| IBIS file stm32u535_545_ufbga100.ibs
[IBIS ver] 4.2
[File name] stm32u535_545_ufbga100.ibs
[File Rev] rev1.0
[Date]  11-09-2023
[Source] Data Created at STMicroelectronics
[Notes]  File originated from ELDO simulations.
[Disclaimer]  This information is for modeling purpose only and is
   not guaranteed. The information is subject to change without
   notice.
[Copyright] Copyright 2023 STMicroelectronics Inc.
|   Component stm32u535_545_ufbga100
[Component] stm32u535_545_ufbga100
[Manufacturer] STMicroelectronics
[Package]
| variable   typ   min   max
R_pkg  0  NA  NA
L_pkg  0  NA  NA
C_pkg  0  NA  NA
[Pin]   signal_name   model_name
A1  PE3  io8_100m_hslv_tamp_ft
A2  PE1  io8_100m_hslv_ft
A3  PB8  io8_100m_hslv_i2c_ft
A4  PH3-BOOT0  io8_100m_ft
A5  PD7  io8_100m_hslv_ft
A6  PD5  io8_100m_hslv_ft
A7  PB4  io8_100m_i2c_ft
A8  PB3  io8_100m_i2c_ft
A9  PA15  io8_100m_ft
A10  PA14  io8_100m_ft
A11  PA13  io8_100m_ft
A12  PA12  io8_usb_ft
B1  PE4  io8_100m_hslv_tamp_ft
B2  PE2  io8_100m_hslv_ft
B3  PB9  io8_100m_hslv_i2c_ft
B4  PB7  io8_166m_hslv_i2c_ft
B5  PB6  io8_100m_i2c_ft
B6  PD6  io8_166m_hslv_ft
B7  PD4  io8_100m_hslv_ft
B8  PD3  io8_166m_hslv_ft
B9  PD1  io8_100m_hslv_ft
B10  PC12  io8_166m_hslv_ft
B11  PC10  io8_100m_hslv_ft
B12  PA11  io8_usb_ft
C1  PC13  io8_100m_ft_v33
C2  PE5  io8_100m_hslv_tamp_ft
C3  PE0  io8_100m_hslv_ft
C4  VDD  power
C5  PB5  io8_166m_hslv_ft
C8  PD2  io8_100m_hslv_ft
C9  PD0  io8_100m_hslv_ft
C10  PC11  io8_100m_hslv_ft
C11  VDDUSB  power
C12  PA10  io8_100m_ft
D1  PC14-OSC32_IN  io8_100m_tamp_ft
D2  PE6  io8_100m_hslv_tamp_ft
D3  VSS  gnd
D10  PA9  io8_100m_ft
D11  PA8  io8_166m_hslv_ft
D12  PC9  io8_100m_hslv_ft
E1  PC15-OSC32_OUT  io8_100m_tamp_ft
E2  VBAT  power
E3  VSS  gnd
E10  PC8  io8_100m_hslv_ft
E11  PC7  io8_100m_hslv_ft
E12  PC6  io8_100m_hslv_ft
F1  PH0-OSC_IN   io8_100m_ft
F2  VSS  gnd
F11  VSS  gnd
F12  VSS  gnd
G1  PH1-OSC_OUT   io8_100m_ft
G2  VDD  power
G11  VDD  power
G12  VDD  power
H1  PC0  io8_100m_hslv_i2c_ft
H2  NRST  nc
H3  VDD  power
H10  PD15  io8_100m_hslv_ft
H11  PD14  io8_100m_hslv_ft
H12  PD13  io8_100m_hslv_i2c_ft
J1  VSSA  nc
J2  PC1  io8_166m_hslv_i2c_ft
J3  PC2  io8_100m_hslv_ft
J10  PD12  io8_100m_hslv_i2c_ft
J11  PD11  io8_100m_hslv_ft
J12  PD10  io8_100m_hslv_ft
K1  VREFM  nc
K2  PC3  io8_100m_hslv_ft
K3  PA2  io8_100m_hslv_ft
K4  PA5  io8_100m_ft
K5  PC4  io8_100m_hslv_ft
K8  PD9  io8_100m_hslv_ft
K9  PD8  io8_100m_hslv_ft
K10  PB15  io8_100m_ft
K11  PB14  io8_100m_i2c_ft
K12  PB13  io8_100m_i2c_ft
L1  VREFP  nc
L2  PA0  io8_100m_hslv_tamp_ft
L3  PA3  io8_166m_hslv_ft
L4  PA6  io8_100m_hslv_ft
L5  PC5  io8_100m_tamp_ft
L6  PB2  io8_100m_hslv_tamp_ft
L7  PE8  io8_100m_hslv_ft
L8  PE10  io8_166m_hslv_ft
L9  PE12  io8_100m_hslv_ft
L10  PB10  io8_166m_hslv_i2c_ft
L11  VCAP  nc
L12  PB12  io8_166m_hslv_ft
M1  VDDA  power
M2  PA1  io8_100m_hslv_tamp_ft
M3  PA4  io8_100m_hslv_ft
M4  PA7  io8_100m_hslv_i2c_ft
M5  PB0  io8_100m_hslv_ft
M6  PB1  io8_100m_hslv_ft
M7  PE7  io8_100m_hslv_ft
M8  PE9  io8_166m_hslv_ft
M9  PE11  io8_100m_hslv_ft
M10  PE13  io8_100m_hslv_ft
M11  PE14  io8_100m_hslv_ft
M12  PE15  io8_100m_hslv_ft
[Package Model]   455-ufbga-7x7-100-ldo-100mhz-230421
[Pin Mapping]   pulldown_ref   pullup_ref   | Comment
A1  gndio  vddiom
A2  gndio  vddiom
A3  gndio  vddiom
A4  gndio  vddiom
A5  gndio  vddiom
A6  gndio  vddiom
A7  gndio  vddiom
A8  gndio  vddiom
A9  gndio  vddiom
A10  gndio  vddiom
A11  gndio  vddiom  | Depending on IO usage
| A11  gndio  vddusb  | Depending on IO usage
A12  gndio  vddiom  | Depending on IO usage
| A12  gndio  vddusb  | Depending on IO usage
B1  gndio  vddiom
B2  gndio  vddiom
B3  gndio  vddiom
B4  gndio  vddiom
B5  gndio  vddiom
B6  gndio  vddiom
B7  gndio  vddiom
B8  gndio  vddiom
B9  gndio  vddiom
B10  gndio  vddiom
B11  gndio  vddiom
B12  gndio  vddiom  | Depending on IO usage
| B12  gndio  vddusb  | Depending on IO usage
C1  gndio  vddiom  | Depending on IO usage
| C1  gndio  vsw  | Depending on IO usage
C2  gndio  vddiom
C3  gndio  vddiom
C4  nc  vddiom
C5  gndio  vddiom
C8  gndio  vddiom
C9  gndio  vddiom
C10  gndio  vddiom
C11  nc  vddusb
C12  gndio  vddiom  | Depending on IO usage
| C12  gndio  vddusb  | Depending on IO usage
D1  gndio  vddiom  | Depending on IO usage
| D1  gndio  vsw  | Depending on IO usage
D2  gndio  vddiom
D3  gndio  nc
D10  gndio  vddiom  | Depending on IO usage
| D10  gndio  vddusb  | Depending on IO usage
D11  gndio  vddiom
D12  gndio  vddiom
E1  gndio  vddiom  | Depending on IO usage
| E1  gndio  vsw  | Depending on IO usage
E2  nc  vsw
E3  gndio  nc
E10  gndio  vddiom
E11  gndio  vddiom
E12  gndio  vddiom
F1  gndio  vddiom
F2  gndio  nc
F11  gndio  nc
F12  gndio  nc
G1  gndio  vddiom
G2  nc  vddiom
G11  nc  vddiom
G12  nc  vddiom
H1  gndio  vddiom
H2  nc   nc
H3  nc  vddiom
H10  gndio  vddiom
H11  gndio  vddiom
H12  gndio  vddiom
J1  nc  nc
J2  gndio  vddiom
J3  gndio  vddiom
J10  gndio  vddiom
J11  gndio  vddiom
J12  gndio  vddiom
K1  nc  nc
K2  gndio  vddiom
K3  gndio  vddiom
K4  gndio  vddiom
K5  gndio  vddiom
K8  gndio  vddiom
K9  gndio  vddiom
K10  gndio  vddiom
K11  gndio  vddiom
K12  gndio  vddiom
L1  nc  nc
L2  gndio  vddiom
L3  gndio  vddiom
L4  gndio  vddiom
L5  gndio  vddiom
L6  gndio  vddiom
L7  gndio  vddiom
L8  gndio  vddiom
L9  gndio  vddiom
L10  gndio  vddiom
L11  nc  nc
L12  gndio  vddiom
M1  nc  vddiom
M2  gndio  vddiom
M3  gndio  vddiom
M4  gndio  vddiom
M5  gndio  vddiom
M6  gndio  vddiom
M7  gndio  vddiom
M8  gndio  vddiom
M9  gndio  vddiom
M10  gndio  vddiom
M11  gndio  vddiom
M12  gndio  vddiom
[Model Selector] io8_100m_ft
io8_100m_ft_hs_1v2  "IO8_FT 100MHz high speed @ 1.2V"
io8_100m_ft_fs_1v2  "IO8_FT 100MHz fast speed @ 1.2V"
io8_100m_ft_fs_pd_1v2  "IO8_FT 100MHz fast speed @ 1.2V pulldown"
io8_100m_ft_ms_1v2  "IO8_FT 100MHz med speed @ 1.2V"
io8_100m_ft_ms_pd_1v2  "IO8_FT 100MHz med speed @ 1.2V pulldown"
io8_100m_ft_ls_1v2  "IO8_FT 100MHz low speed @ 1.2V"
io8_100m_ft_ls_pd_1v2  "IO8_FT 100MHz low speed @ 1.2V pulldown"
io8_100m_ft_hs_1v8  "IO8_FT 100MHz high speed @ 1.8V"
io8_100m_ft_hs_pd_1v8  "IO8_FT 100MHz high speed @ 1.8V pulldown"
io8_100m_ft_fs_1v8  "IO8_FT 100MHz fast speed @ 1.8V"
io8_100m_ft_fs_pd_1v8  "IO8_FT 100MHz fast speed @ 1.8V pulldown"
io8_100m_ft_ms_1v8  "IO8_FT 100MHz med speed @ 1.8V"
io8_100m_ft_ms_pd_1v8  "IO8_FT 100MHz med speed @ 1.8V pulldown"
io8_100m_ft_ls_1v8  "IO8_FT 100MHz low speed @ 1.8V"
io8_100m_ft_ls_pd_1v8  "IO8_FT 100MHz low speed @ 1.8V pulldown"
io8_100m_ft_hs_3v3  "IO8_FT 100MHz high speed @ 3.3V"
io8_100m_ft_hs_pd_3v3  "IO8_FT 100MHz high speed @ 3.3V pulldown"
io8_100m_ft_fs_3v3  "IO8_FT 100MHz fast speed @ 3.3V"
io8_100m_ft_fs_pd_3v3  "IO8_FT 100MHz fast speed @ 3.3V pulldown"
io8_100m_ft_ms_3v3  "IO8_FT 100MHz med speed @ 3.3V"
io8_100m_ft_ms_pd_3v3  "IO8_FT 100MHz med speed @ 3.3V pulldown"
io8_100m_ft_ls_3v3  "IO8_FT 100MHz low speed @ 3.3V"
io8_100m_ft_ls_pd_3v3  "IO8_FT 100MHz low speed @ 3.3V pulldown"
[Model Selector] io8_100m_hslv_ft
io8_100m_ft_hs_1v2  "IO8_FT 100MHz high speed @ 1.2V"
io8_100m_ft_hs_pu_1v2  "IO8_FT 100MHz high speed @ 1.2V pullup"
io8_100m_ft_hs_pd_1v2  "IO8_FT 100MHz high speed @ 1.2V pulldown"
io8_100m_ft_fs_1v2  "IO8_FT 100MHz fast speed @ 1.2V"
io8_100m_ft_fs_pu_1v2  "IO8_FT 100MHz fast speed @ 1.2V pullup"
io8_100m_ft_fs_pd_1v2  "IO8_FT 100MHz fast speed @ 1.2V pulldown"
io8_100m_ft_ms_1v2  "IO8_FT 100MHz med speed @ 1.2V"
io8_100m_ft_ms_pu_1v2  "IO8_FT 100MHz med speed @ 1.2V pullup"
io8_100m_ft_ms_pd_1v2  "IO8_FT 100MHz med speed @ 1.2V pulldown"
io8_100m_ft_ls_1v2  "IO8_FT 100MHz low speed @ 1.2V"
io8_100m_ft_ls_pu_1v2  "IO8_FT 100MHz low speed @ 1.2V pullup"
io8_100m_ft_ls_pd_1v2  "IO8_FT 100MHz low speed @ 1.2V pulldown"
io8_100m_ft_hs_1v8  "IO8_FT 100MHz high speed @ 1.8V"
io8_100m_ft_hs_pu_1v8  "IO8_FT 100MHz high speed @ 1.8V pullup"
io8_100m_ft_hs_pd_1v8  "IO8_FT 100MHz high speed @ 1.8V pulldown"
io8_100m_ft_fs_1v8  "IO8_FT 100MHz fast speed @ 1.8V"
io8_100m_ft_fs_pu_1v8  "IO8_FT 100MHz fast speed @ 1.8V pullup"
io8_100m_ft_fs_pd_1v8  "IO8_FT 100MHz fast speed @ 1.8V pulldown"
io8_100m_ft_ms_1v8  "IO8_FT 100MHz med speed @ 1.8V"
io8_100m_ft_ms_pu_1v8  "IO8_FT 100MHz med speed @ 1.8V pullup"
io8_100m_ft_ms_pd_1v8  "IO8_FT 100MHz med speed @ 1.8V pulldown"
io8_100m_ft_ls_1v8  "IO8_FT 100MHz low speed @ 1.8V"
io8_100m_ft_ls_pu_1v8  "IO8_FT 100MHz low speed @ 1.8V pullup"
io8_100m_ft_ls_pd_1v8  "IO8_FT 100MHz low speed @ 1.8V pulldown"
io8_100m_ft_hs_3v3  "IO8_FT 100MHz high speed @ 3.3V"
io8_100m_ft_hs_pu_3v3  "IO8_FT 100MHz high speed @ 3.3V pullup"
io8_100m_ft_hs_pd_3v3  "IO8_FT 100MHz high speed @ 3.3V pulldown"
io8_100m_ft_fs_3v3  "IO8_FT 100MHz fast speed @ 3.3V"
io8_100m_ft_fs_pu_3v3  "IO8_FT 100MHz fast speed @ 3.3V pullup"
io8_100m_ft_fs_pd_3v3  "IO8_FT 100MHz fast speed @ 3.3V pulldown"
io8_100m_ft_ms_3v3  "IO8_FT 100MHz med speed @ 3.3V"
io8_100m_ft_ms_pu_3v3  "IO8_FT 100MHz med speed @ 3.3V pullup"
io8_100m_ft_ms_pd_3v3  "IO8_FT 100MHz med speed @ 3.3V pulldown"
io8_100m_ft_ls_3v3  "IO8_FT 100MHz low speed @ 3.3V"
io8_100m_ft_ls_pu_3v3  "IO8_FT 100MHz low speed @ 3.3V pullup"
io8_100m_ft_ls_pd_3v3  "IO8_FT 100MHz low speed @ 3.3V pulldown"
io8_100m_hslv_ft_hs_1v2  "IO8_FT 100MHz HSLV high speed @ 1.2V"
io8_100m_hslv_ft_hs_pu_1v2  "IO8_FT 100MHz HSLV high speed @ 1.2V pullup"
io8_100m_hslv_ft_hs_pd_1v2  "IO8_FT 100MHz HSLV high speed @ 1.2V pulldown"
io8_100m_hslv_ft_fs_1v2  "IO8_FT 100MHz HSLV fast speed @ 1.2V"
io8_100m_hslv_ft_fs_pu_1v2  "IO8_FT 100MHz HSLV fast speed @ 1.2V pullup"
io8_100m_hslv_ft_fs_pd_1v2  "IO8_FT 100MHz HSLV fast speed @ 1.2V pulldown"
io8_100m_hslv_ft_ms_1v2  "IO8_FT 100MHz HSLV med speed @ 1.2V"
io8_100m_hslv_ft_ms_pu_1v2  "IO8_FT 100MHz HSLV med speed @ 1.2V pullup"
io8_100m_hslv_ft_ms_pd_1v2  "IO8_FT 100MHz HSLV med speed @ 1.2V pulldown"
io8_100m_hslv_ft_ls_1v2  "IO8_FT 100MHz HSLV low speed @ 1.2V"
io8_100m_hslv_ft_ls_pu_1v2  "IO8_FT 100MHz HSLV low speed @ 1.2V pullup"
io8_100m_hslv_ft_ls_pd_1v2  "IO8_FT 100MHz HSLV low speed @ 1.2V pulldown"
io8_100m_hslv_ft_hs_1v8  "IO8_FT 100MHz HSLV high speed @ 1.8V"
io8_100m_hslv_ft_hs_pu_1v8  "IO8_FT 100MHz HSLV high speed @ 1.8V pullup"
io8_100m_hslv_ft_hs_pd_1v8  "IO8_FT 100MHz HSLV high speed @ 1.8V pulldown"
io8_100m_hslv_ft_fs_1v8  "IO8_FT 100MHz HSLV fast speed @ 1.8V"
io8_100m_hslv_ft_fs_pu_1v8  "IO8_FT 100MHz HSLV fast speed @ 1.8V pullup"
io8_100m_hslv_ft_fs_pd_1v8  "IO8_FT 100MHz HSLV fast speed @ 1.8V pulldown"
io8_100m_hslv_ft_ms_1v8  "IO8_FT 100MHz HSLV med speed @ 1.8V"
io8_100m_hslv_ft_ms_pu_1v8  "IO8_FT 100MHz HSLV med speed @ 1.8V pullup"
io8_100m_hslv_ft_ms_pd_1v8  "IO8_FT 100MHz HSLV med speed @ 1.8V pulldown"
io8_100m_hslv_ft_ls_1v8  "IO8_FT 100MHz HSLV low speed @ 1.8V"
io8_100m_hslv_ft_ls_pu_1v8  "IO8_FT 100MHz HSLV low speed @ 1.8V pullup"
io8_100m_hslv_ft_ls_pd_1v8  "IO8_FT 100MHz HSLV low speed @ 1.8V pulldown"
io8_100m_hslv_ft_hs_2v5  "IO8_FT 100MHz HSLV high speed @ 2.5V"
io8_100m_hslv_ft_hs_pu_2v5  "IO8_FT 100MHz HSLV high speed @ 2.5V pullup"
io8_100m_hslv_ft_hs_pd_2v5  "IO8_FT 100MHz HSLV high speed @ 2.5V pulldown"
io8_100m_hslv_ft_fs_2v5  "IO8_FT 100MHz HSLV fast speed @ 2.5V"
io8_100m_hslv_ft_fs_pu_2v5  "IO8_FT 100MHz HSLV fast speed @ 2.5V pullup"
io8_100m_hslv_ft_fs_pd_2v5  "IO8_FT 100MHz HSLV fast speed @ 2.5V pulldown"
io8_100m_hslv_ft_ms_2v5  "IO8_FT 100MHz HSLV med speed @ 2.5V"
io8_100m_hslv_ft_ms_pu_2v5  "IO8_FT 100MHz HSLV med speed @ 2.5V pullup"
io8_100m_hslv_ft_ms_pd_2v5  "IO8_FT 100MHz HSLV med speed @ 2.5V pulldown"
io8_100m_hslv_ft_ls_2v5  "IO8_FT 100MHz HSLV low speed @ 2.5V"
io8_100m_hslv_ft_ls_pu_2v5  "IO8_FT 100MHz HSLV low speed @ 2.5V pullup"
io8_100m_hslv_ft_ls_pd_2v5  "IO8_FT 100MHz HSLV low speed @ 2.5V pulldown"
[Model Selector] io8_100m_hslv_i2c_ft
io8_100m_ft_hs_1v2  "IO8_FT 100MHz high speed @ 1.2V"
io8_100m_ft_hs_pu_1v2  "IO8_FT 100MHz high speed @ 1.2V pullup"
io8_100m_ft_hs_pd_1v2  "IO8_FT 100MHz high speed @ 1.2V pulldown"
io8_100m_ft_fs_1v2  "IO8_FT 100MHz fast speed @ 1.2V"
io8_100m_ft_fs_pu_1v2  "IO8_FT 100MHz fast speed @ 1.2V pullup"
io8_100m_ft_fs_pd_1v2  "IO8_FT 100MHz fast speed @ 1.2V pulldown"
io8_100m_ft_ms_1v2  "IO8_FT 100MHz med speed @ 1.2V"
io8_100m_ft_ms_pu_1v2  "IO8_FT 100MHz med speed @ 1.2V pullup"
io8_100m_ft_ms_pd_1v2  "IO8_FT 100MHz med speed @ 1.2V pulldown"
io8_100m_ft_ls_1v2  "IO8_FT 100MHz low speed @ 1.2V"
io8_100m_ft_ls_pu_1v2  "IO8_FT 100MHz low speed @ 1.2V pullup"
io8_100m_ft_ls_pd_1v2  "IO8_FT 100MHz low speed @ 1.2V pulldown"
io8_100m_ft_hs_1v8  "IO8_FT 100MHz high speed @ 1.8V"
io8_100m_ft_hs_pu_1v8  "IO8_FT 100MHz high speed @ 1.8V pullup"
io8_100m_ft_hs_pd_1v8  "IO8_FT 100MHz high speed @ 1.8V pulldown"
io8_100m_ft_fs_1v8  "IO8_FT 100MHz fast speed @ 1.8V"
io8_100m_ft_fs_pu_1v8  "IO8_FT 100MHz fast speed @ 1.8V pullup"
io8_100m_ft_fs_pd_1v8  "IO8_FT 100MHz fast speed @ 1.8V pulldown"
io8_100m_ft_ms_1v8  "IO8_FT 100MHz med speed @ 1.8V"
io8_100m_ft_ms_pu_1v8  "IO8_FT 100MHz med speed @ 1.8V pullup"
io8_100m_ft_ms_pd_1v8  "IO8_FT 100MHz med speed @ 1.8V pulldown"
io8_100m_ft_ls_1v8  "IO8_FT 100MHz low speed @ 1.8V"
io8_100m_ft_ls_pu_1v8  "IO8_FT 100MHz low speed @ 1.8V pullup"
io8_100m_ft_ls_pd_1v8  "IO8_FT 100MHz low speed @ 1.8V pulldown"
io8_100m_ft_hs_3v3  "IO8_FT 100MHz high speed @ 3.3V"
io8_100m_ft_hs_pu_3v3  "IO8_FT 100MHz high speed @ 3.3V pullup"
io8_100m_ft_hs_pd_3v3  "IO8_FT 100MHz high speed @ 3.3V pulldown"
io8_100m_ft_fs_3v3  "IO8_FT 100MHz fast speed @ 3.3V"
io8_100m_ft_fs_pu_3v3  "IO8_FT 100MHz fast speed @ 3.3V pullup"
io8_100m_ft_fs_pd_3v3  "IO8_FT 100MHz fast speed @ 3.3V pulldown"
io8_100m_ft_ms_3v3  "IO8_FT 100MHz med speed @ 3.3V"
io8_100m_ft_ms_pu_3v3  "IO8_FT 100MHz med speed @ 3.3V pullup"
io8_100m_ft_ms_pd_3v3  "IO8_FT 100MHz med speed @ 3.3V pulldown"
io8_100m_ft_ls_3v3  "IO8_FT 100MHz low speed @ 3.3V"
io8_100m_ft_ls_pu_3v3  "IO8_FT 100MHz low speed @ 3.3V pullup"
io8_100m_ft_ls_pd_3v3  "IO8_FT 100MHz low speed @ 3.3V pulldown"
io8_100m_hslv_ft_hs_1v2  "IO8_FT 100MHz HSLV high speed @ 1.2V"
io8_100m_hslv_ft_hs_pu_1v2  "IO8_FT 100MHz HSLV high speed @ 1.2V pullup"
io8_100m_hslv_ft_hs_pd_1v2  "IO8_FT 100MHz HSLV high speed @ 1.2V pulldown"
io8_100m_hslv_ft_fs_1v2  "IO8_FT 100MHz HSLV fast speed @ 1.2V"
io8_100m_hslv_ft_fs_pu_1v2  "IO8_FT 100MHz HSLV fast speed @ 1.2V pullup"
io8_100m_hslv_ft_fs_pd_1v2  "IO8_FT 100MHz HSLV fast speed @ 1.2V pulldown"
io8_100m_hslv_ft_ms_1v2  "IO8_FT 100MHz HSLV med speed @ 1.2V"
io8_100m_hslv_ft_ms_pu_1v2  "IO8_FT 100MHz HSLV med speed @ 1.2V pullup"
io8_100m_hslv_ft_ms_pd_1v2  "IO8_FT 100MHz HSLV med speed @ 1.2V pulldown"
io8_100m_hslv_ft_ls_1v2  "IO8_FT 100MHz HSLV low speed @ 1.2V"
io8_100m_hslv_ft_ls_pu_1v2  "IO8_FT 100MHz HSLV low speed @ 1.2V pullup"
io8_100m_hslv_ft_ls_pd_1v2  "IO8_FT 100MHz HSLV low speed @ 1.2V pulldown"
io8_100m_hslv_ft_hs_1v8  "IO8_FT 100MHz HSLV high speed @ 1.8V"
io8_100m_hslv_ft_hs_pu_1v8  "IO8_FT 100MHz HSLV high speed @ 1.8V pullup"
io8_100m_hslv_ft_hs_pd_1v8  "IO8_FT 100MHz HSLV high speed @ 1.8V pulldown"
io8_100m_hslv_ft_fs_1v8  "IO8_FT 100MHz HSLV fast speed @ 1.8V"
io8_100m_hslv_ft_fs_pu_1v8  "IO8_FT 100MHz HSLV fast speed @ 1.8V pullup"
io8_100m_hslv_ft_fs_pd_1v8  "IO8_FT 100MHz HSLV fast speed @ 1.8V pulldown"
io8_100m_hslv_ft_ms_1v8  "IO8_FT 100MHz HSLV med speed @ 1.8V"
io8_100m_hslv_ft_ms_pu_1v8  "IO8_FT 100MHz HSLV med speed @ 1.8V pullup"
io8_100m_hslv_ft_ms_pd_1v8  "IO8_FT 100MHz HSLV med speed @ 1.8V pulldown"
io8_100m_hslv_ft_ls_1v8  "IO8_FT 100MHz HSLV low speed @ 1.8V"
io8_100m_hslv_ft_ls_pu_1v8  "IO8_FT 100MHz HSLV low speed @ 1.8V pullup"
io8_100m_hslv_ft_ls_pd_1v8  "IO8_FT 100MHz HSLV low speed @ 1.8V pulldown"
io8_100m_hslv_ft_hs_2v5  "IO8_FT 100MHz HSLV high speed @ 2.5V"
io8_100m_hslv_ft_hs_pu_2v5  "IO8_FT 100MHz HSLV high speed @ 2.5V pullup"
io8_100m_hslv_ft_hs_pd_2v5  "IO8_FT 100MHz HSLV high speed @ 2.5V pulldown"
io8_100m_hslv_ft_fs_2v5  "IO8_FT 100MHz HSLV fast speed @ 2.5V"
io8_100m_hslv_ft_fs_pu_2v5  "IO8_FT 100MHz HSLV fast speed @ 2.5V pullup"
io8_100m_hslv_ft_fs_pd_2v5  "IO8_FT 100MHz HSLV fast speed @ 2.5V pulldown"
io8_100m_hslv_ft_ms_2v5  "IO8_FT 100MHz HSLV med speed @ 2.5V"
io8_100m_hslv_ft_ms_pu_2v5  "IO8_FT 100MHz HSLV med speed @ 2.5V pullup"
io8_100m_hslv_ft_ms_pd_2v5  "IO8_FT 100MHz HSLV med speed @ 2.5V pulldown"
io8_100m_hslv_ft_ls_2v5  "IO8_FT 100MHz HSLV low speed @ 2.5V"
io8_100m_hslv_ft_ls_pu_2v5  "IO8_FT 100MHz HSLV low speed @ 2.5V pullup"
io8_100m_hslv_ft_ls_pd_2v5  "IO8_FT 100MHz HSLV low speed @ 2.5V pulldown"
[Model Selector] io8_100m_hslv_tamp_ft
io8_100m_ft_hs_1v2  "IO8_FT 100MHz high speed @ 1.2V"
io8_100m_ft_hs_pu_1v2  "IO8_FT 100MHz high speed @ 1.2V pullup"
io8_100m_ft_hs_pd_1v2  "IO8_FT 100MHz high speed @ 1.2V pulldown"
io8_100m_ft_fs_1v2  "IO8_FT 100MHz fast speed @ 1.2V"
io8_100m_ft_fs_pu_1v2  "IO8_FT 100MHz fast speed @ 1.2V pullup"
io8_100m_ft_fs_pd_1v2  "IO8_FT 100MHz fast speed @ 1.2V pulldown"
io8_100m_ft_ms_1v2  "IO8_FT 100MHz med speed @ 1.2V"
io8_100m_ft_ms_pu_1v2  "IO8_FT 100MHz med speed @ 1.2V pullup"
io8_100m_ft_ms_pd_1v2  "IO8_FT 100MHz med speed @ 1.2V pulldown"
io8_100m_ft_ls_1v2  "IO8_FT 100MHz low speed @ 1.2V"
io8_100m_ft_ls_pu_1v2  "IO8_FT 100MHz low speed @ 1.2V pullup"
io8_100m_ft_ls_pd_1v2  "IO8_FT 100MHz low speed @ 1.2V pulldown"
io8_100m_ft_hs_1v8  "IO8_FT 100MHz high speed @ 1.8V"
io8_100m_ft_hs_pu_1v8  "IO8_FT 100MHz high speed @ 1.8V pullup"
io8_100m_ft_hs_pd_1v8  "IO8_FT 100MHz high speed @ 1.8V pulldown"
io8_100m_ft_fs_1v8  "IO8_FT 100MHz fast speed @ 1.8V"
io8_100m_ft_fs_pu_1v8  "IO8_FT 100MHz fast speed @ 1.8V pullup"
io8_100m_ft_fs_pd_1v8  "IO8_FT 100MHz fast speed @ 1.8V pulldown"
io8_100m_ft_ms_1v8  "IO8_FT 100MHz med speed @ 1.8V"
io8_100m_ft_ms_pu_1v8  "IO8_FT 100MHz med speed @ 1.8V pullup"
io8_100m_ft_ms_pd_1v8  "IO8_FT 100MHz med speed @ 1.8V pulldown"
io8_100m_ft_ls_1v8  "IO8_FT 100MHz low speed @ 1.8V"
io8_100m_ft_ls_pu_1v8  "IO8_FT 100MHz low speed @ 1.8V pullup"
io8_100m_ft_ls_pd_1v8  "IO8_FT 100MHz low speed @ 1.8V pulldown"
io8_100m_ft_hs_3v3  "IO8_FT 100MHz high speed @ 3.3V"
io8_100m_ft_hs_pu_3v3  "IO8_FT 100MHz high speed @ 3.3V pullup"
io8_100m_ft_hs_pd_3v3  "IO8_FT 100MHz high speed @ 3.3V pulldown"
io8_100m_ft_fs_3v3  "IO8_FT 100MHz fast speed @ 3.3V"
io8_100m_ft_fs_pu_3v3  "IO8_FT 100MHz fast speed @ 3.3V pullup"
io8_100m_ft_fs_pd_3v3  "IO8_FT 100MHz fast speed @ 3.3V pulldown"
io8_100m_ft_ms_3v3  "IO8_FT 100MHz med speed @ 3.3V"
io8_100m_ft_ms_pu_3v3  "IO8_FT 100MHz med speed @ 3.3V pullup"
io8_100m_ft_ms_pd_3v3  "IO8_FT 100MHz med speed @ 3.3V pulldown"
io8_100m_ft_ls_3v3  "IO8_FT 100MHz low speed @ 3.3V"
io8_100m_ft_ls_pu_3v3  "IO8_FT 100MHz low speed @ 3.3V pullup"
io8_100m_ft_ls_pd_3v3  "IO8_FT 100MHz low speed @ 3.3V pulldown"
io8_100m_hslv_ft_hs_1v2  "IO8_FT 100MHz HSLV high speed @ 1.2V"
io8_100m_hslv_ft_hs_pu_1v2  "IO8_FT 100MHz HSLV high speed @ 1.2V pullup"
io8_100m_hslv_ft_hs_pd_1v2  "IO8_FT 100MHz HSLV high speed @ 1.2V pulldown"
io8_100m_hslv_ft_fs_1v2  "IO8_FT 100MHz HSLV fast speed @ 1.2V"
io8_100m_hslv_ft_fs_pu_1v2  "IO8_FT 100MHz HSLV fast speed @ 1.2V pullup"
io8_100m_hslv_ft_fs_pd_1v2  "IO8_FT 100MHz HSLV fast speed @ 1.2V pulldown"
io8_100m_hslv_ft_ms_1v2  "IO8_FT 100MHz HSLV med speed @ 1.2V"
io8_100m_hslv_ft_ms_pu_1v2  "IO8_FT 100MHz HSLV med speed @ 1.2V pullup"
io8_100m_hslv_ft_ms_pd_1v2  "IO8_FT 100MHz HSLV med speed @ 1.2V pulldown"
io8_100m_hslv_ft_ls_1v2  "IO8_FT 100MHz HSLV low speed @ 1.2V"
io8_100m_hslv_ft_ls_pu_1v2  "IO8_FT 100MHz HSLV low speed @ 1.2V pullup"
io8_100m_hslv_ft_ls_pd_1v2  "IO8_FT 100MHz HSLV low speed @ 1.2V pulldown"
io8_100m_hslv_ft_hs_1v8  "IO8_FT 100MHz HSLV high speed @ 1.8V"
io8_100m_hslv_ft_hs_pu_1v8  "IO8_FT 100MHz HSLV high speed @ 1.8V pullup"
io8_100m_hslv_ft_hs_pd_1v8  "IO8_FT 100MHz HSLV high speed @ 1.8V pulldown"
io8_100m_hslv_ft_fs_1v8  "IO8_FT 100MHz HSLV fast speed @ 1.8V"
io8_100m_hslv_ft_fs_pu_1v8  "IO8_FT 100MHz HSLV fast speed @ 1.8V pullup"
io8_100m_hslv_ft_fs_pd_1v8  "IO8_FT 100MHz HSLV fast speed @ 1.8V pulldown"
io8_100m_hslv_ft_ms_1v8  "IO8_FT 100MHz HSLV med speed @ 1.8V"
io8_100m_hslv_ft_ms_pu_1v8  "IO8_FT 100MHz HSLV med speed @ 1.8V pullup"
io8_100m_hslv_ft_ms_pd_1v8  "IO8_FT 100MHz HSLV med speed @ 1.8V pulldown"
io8_100m_hslv_ft_ls_1v8  "IO8_FT 100MHz HSLV low speed @ 1.8V"
io8_100m_hslv_ft_ls_pu_1v8  "IO8_FT 100MHz HSLV low speed @ 1.8V pullup"
io8_100m_hslv_ft_ls_pd_1v8  "IO8_FT 100MHz HSLV low speed @ 1.8V pulldown"
io8_100m_hslv_ft_hs_2v5  "IO8_FT 100MHz HSLV high speed @ 2.5V"
io8_100m_hslv_ft_hs_pu_2v5  "IO8_FT 100MHz HSLV high speed @ 2.5V pullup"
io8_100m_hslv_ft_hs_pd_2v5  "IO8_FT 100MHz HSLV high speed @ 2.5V pulldown"
io8_100m_hslv_ft_fs_2v5  "IO8_FT 100MHz HSLV fast speed @ 2.5V"
io8_100m_hslv_ft_fs_pu_2v5  "IO8_FT 100MHz HSLV fast speed @ 2.5V pullup"
io8_100m_hslv_ft_fs_pd_2v5  "IO8_FT 100MHz HSLV fast speed @ 2.5V pulldown"
io8_100m_hslv_ft_ms_2v5  "IO8_FT 100MHz HSLV med speed @ 2.5V"
io8_100m_hslv_ft_ms_pu_2v5  "IO8_FT 100MHz HSLV med speed @ 2.5V pullup"
io8_100m_hslv_ft_ms_pd_2v5  "IO8_FT 100MHz HSLV med speed @ 2.5V pulldown"
io8_100m_hslv_ft_ls_2v5  "IO8_FT 100MHz HSLV low speed @ 2.5V"
io8_100m_hslv_ft_ls_pu_2v5  "IO8_FT 100MHz HSLV low speed @ 2.5V pullup"
io8_100m_hslv_ft_ls_pd_2v5  "IO8_FT 100MHz HSLV low speed @ 2.5V pulldown"
io8_ft_v33_hs_1v2  "IO8_FT_V33 high speed @ 1.2V"
io8_ft_v33_hs_pu_1v2  "IO8_FT_V33 high speed @ 1.2V pullup"
io8_ft_v33_hs_pd_1v2  "IO8_FT_V33 high speed @ 1.2V pulldown"
io8_ft_v33_fs_1v2  "IO8_FT_V33 fast speed @ 1.2V"
io8_ft_v33_fs_pu_1v2  "IO8_FT_V33 fast speed @ 1.2V pullup"
io8_ft_v33_fs_pd_1v2  "IO8_FT_V33 fast speed @ 1.2V pulldown"
io8_ft_v33_ms_1v2  "IO8_FT_V33 med speed @ 1.2V"
io8_ft_v33_ms_pu_1v2  "IO8_FT_V33 med speed @ 1.2V pullup"
io8_ft_v33_ms_pd_1v2  "IO8_FT_V33 med speed @ 1.2V pulldown"
io8_ft_v33_ls_1v2  "IO8_FT_V33 low speed @ 1.2V"
io8_ft_v33_ls_pu_1v2  "IO8_FT_V33 low speed @ 1.2V pullup"
io8_ft_v33_ls_pd_1v2  "IO8_FT_V33 low speed @ 1.2V pulldown"
io8_ft_v33_hs_1v8  "IO8_FT_V33 high speed @ 1.8V"
io8_ft_v33_hs_pu_1v8  "IO8_FT_V33 high speed @ 1.8V pullup"
io8_ft_v33_hs_pd_1v8  "IO8_FT_V33 high speed @ 1.8V pulldown"
io8_ft_v33_fs_1v8  "IO8_FT_V33 fast speed @ 1.8V"
io8_ft_v33_fs_pu_1v8  "IO8_FT_V33 fast speed @ 1.8V pullup"
io8_ft_v33_fs_pd_1v8  "IO8_FT_V33 fast speed @ 1.8V pulldown"
io8_ft_v33_ms_1v8  "IO8_FT_V33 med speed @ 1.8V"
io8_ft_v33_ms_pu_1v8  "IO8_FT_V33 med speed @ 1.8V pullup"
io8_ft_v33_ms_pd_1v8  "IO8_FT_V33 med speed @ 1.8V pulldown"
io8_ft_v33_ls_1v8  "IO8_FT_V33 low speed @ 1.8V"
io8_ft_v33_ls_pu_1v8  "IO8_FT_V33 low speed @ 1.8V pullup"
io8_ft_v33_ls_pd_1v8  "IO8_FT_V33 low speed @ 1.8V pulldown"
io8_ft_v33_hs_3v3  "IO8_FT_V33 high speed @ 3.3V"
io8_ft_v33_hs_pu_3v3  "IO8_FT_V33 high speed @ 3.3V pullup"
io8_ft_v33_hs_pd_3v3  "IO8_FT_V33 high speed @ 3.3V pulldown"
io8_ft_v33_fs_3v3  "IO8_FT_V33 fast speed @ 3.3V"
io8_ft_v33_fs_pu_3v3  "IO8_FT_V33 fast speed @ 3.3V pullup"
io8_ft_v33_fs_pd_3v3  "IO8_FT_V33 fast speed @ 3.3V pulldown"
io8_ft_v33_ms_3v3  "IO8_FT_V33 med speed @ 3.3V"
io8_ft_v33_ms_pu_3v3  "IO8_FT_V33 med speed @ 3.3V pullup"
io8_ft_v33_ms_pd_3v3  "IO8_FT_V33 med speed @ 3.3V pulldown"
io8_ft_v33_ls_3v3  "IO8_FT_V33 low speed @ 3.3V"
io8_ft_v33_ls_pu_3v3  "IO8_FT_V33 low speed @ 3.3V pullup"
io8_ft_v33_ls_pd_3v3  "IO8_FT_V33 low speed @ 3.3V pulldown"
[Model Selector] io8_100m_i2c_ft
io8_100m_ft_hs_1v2  "IO8_FT 100MHz high speed @ 1.2V"
io8_100m_ft_hs_pu_1v2  "IO8_FT 100MHz high speed @ 1.2V pullup"
io8_100m_ft_hs_pd_1v2  "IO8_FT 100MHz high speed @ 1.2V pulldown"
io8_100m_ft_fs_1v2  "IO8_FT 100MHz fast speed @ 1.2V"
io8_100m_ft_fs_pu_1v2  "IO8_FT 100MHz fast speed @ 1.2V pullup"
io8_100m_ft_fs_pd_1v2  "IO8_FT 100MHz fast speed @ 1.2V pulldown"
io8_100m_ft_ms_1v2  "IO8_FT 100MHz med speed @ 1.2V"
io8_100m_ft_ms_pu_1v2  "IO8_FT 100MHz med speed @ 1.2V pullup"
io8_100m_ft_ms_pd_1v2  "IO8_FT 100MHz med speed @ 1.2V pulldown"
io8_100m_ft_ls_1v2  "IO8_FT 100MHz low speed @ 1.2V"
io8_100m_ft_ls_pu_1v2  "IO8_FT 100MHz low speed @ 1.2V pullup"
io8_100m_ft_ls_pd_1v2  "IO8_FT 100MHz low speed @ 1.2V pulldown"
io8_100m_ft_hs_1v8  "IO8_FT 100MHz high speed @ 1.8V"
io8_100m_ft_hs_pu_1v8  "IO8_FT 100MHz high speed @ 1.8V pullup"
io8_100m_ft_hs_pd_1v8  "IO8_FT 100MHz high speed @ 1.8V pulldown"
io8_100m_ft_fs_1v8  "IO8_FT 100MHz fast speed @ 1.8V"
io8_100m_ft_fs_pu_1v8  "IO8_FT 100MHz fast speed @ 1.8V pullup"
io8_100m_ft_fs_pd_1v8  "IO8_FT 100MHz fast speed @ 1.8V pulldown"
io8_100m_ft_ms_1v8  "IO8_FT 100MHz med speed @ 1.8V"
io8_100m_ft_ms_pu_1v8  "IO8_FT 100MHz med speed @ 1.8V pullup"
io8_100m_ft_ms_pd_1v8  "IO8_FT 100MHz med speed @ 1.8V pulldown"
io8_100m_ft_ls_1v8  "IO8_FT 100MHz low speed @ 1.8V"
io8_100m_ft_ls_pu_1v8  "IO8_FT 100MHz low speed @ 1.8V pullup"
io8_100m_ft_ls_pd_1v8  "IO8_FT 100MHz low speed @ 1.8V pulldown"
io8_100m_ft_hs_3v3  "IO8_FT 100MHz high speed @ 3.3V"
io8_100m_ft_hs_pu_3v3  "IO8_FT 100MHz high speed @ 3.3V pullup"
io8_100m_ft_hs_pd_3v3  "IO8_FT 100MHz high speed @ 3.3V pulldown"
io8_100m_ft_fs_3v3  "IO8_FT 100MHz fast speed @ 3.3V"
io8_100m_ft_fs_pu_3v3  "IO8_FT 100MHz fast speed @ 3.3V pullup"
io8_100m_ft_fs_pd_3v3  "IO8_FT 100MHz fast speed @ 3.3V pulldown"
io8_100m_ft_ms_3v3  "IO8_FT 100MHz med speed @ 3.3V"
io8_100m_ft_ms_pu_3v3  "IO8_FT 100MHz med speed @ 3.3V pullup"
io8_100m_ft_ms_pd_3v3  "IO8_FT 100MHz med speed @ 3.3V pulldown"
io8_100m_ft_ls_3v3  "IO8_FT 100MHz low speed @ 3.3V"
io8_100m_ft_ls_pu_3v3  "IO8_FT 100MHz low speed @ 3.3V pullup"
io8_100m_ft_ls_pd_3v3  "IO8_FT 100MHz low speed @ 3.3V pulldown"
io8_100m_i2c_ft_1v2  "IO8_FT 100MHz I2C @ 1.2V"
io8_100m_i2c_ft_pu_1v2  "IO8_FT 100MHz I2C @ 1.2V pullup"
io8_100m_i2c_ft_pd_1v2  "IO8_FT 100MHz I2C @ 1.2V pulldown"
io8_100m_i2c_ft_1v8  "IO8_FT 100MHz I2C @ 1.8V"
io8_100m_i2c_ft_pu_1v8  "IO8_FT 100MHz I2C @ 1.8V pullup"
io8_100m_i2c_ft_pd_1v8  "IO8_FT 100MHz I2C @ 1,8V pulldown"
io8_100m_i2c_ft_3v3  "IO8_FT 100MHz I2C @ 3.3V"
io8_100m_i2c_ft_pu_3v3  "IO8_FT 100MHz I2C HSLV @ 3.3V pullup"
io8_100m_i2c_ft_pd_3v3  "IO8_FT 100MHz I2C @ 3.3V pulldown"
[Model Selector] io8_100m_tamp_ft
io8_100m_ft_hs_1v2  "IO8_FT 100MHz high speed @ 1.2V"
io8_100m_ft_hs_pu_1v2  "IO8_FT 100MHz high speed @ 1.2V pullup"
io8_100m_ft_hs_pd_1v2  "IO8_FT 100MHz high speed @ 1.2V pulldown"
io8_100m_ft_fs_1v2  "IO8_FT 100MHz fast speed @ 1.2V"
io8_100m_ft_fs_pu_1v2  "IO8_FT 100MHz fast speed @ 1.2V pullup"
io8_100m_ft_fs_pd_1v2  "IO8_FT 100MHz fast speed @ 1.2V pulldown"
io8_100m_ft_ms_1v2  "IO8_FT 100MHz med speed @ 1.2V"
io8_100m_ft_ms_pu_1v2  "IO8_FT 100MHz med speed @ 1.2V pullup"
io8_100m_ft_ms_pd_1v2  "IO8_FT 100MHz med speed @ 1.2V pulldown"
io8_100m_ft_ls_1v2  "IO8_FT 100MHz low speed @ 1.2V"
io8_100m_ft_ls_pu_1v2  "IO8_FT 100MHz low speed @ 1.2V pullup"
io8_100m_ft_ls_pd_1v2  "IO8_FT 100MHz low speed @ 1.2V pulldown"
io8_100m_ft_hs_1v8  "IO8_FT 100MHz high speed @ 1.8V"
io8_100m_ft_hs_pu_1v8  "IO8_FT 100MHz high speed @ 1.8V pullup"
io8_100m_ft_hs_pd_1v8  "IO8_FT 100MHz high speed @ 1.8V pulldown"
io8_100m_ft_fs_1v8  "IO8_FT 100MHz fast speed @ 1.8V"
io8_100m_ft_fs_pu_1v8  "IO8_FT 100MHz fast speed @ 1.8V pullup"
io8_100m_ft_fs_pd_1v8  "IO8_FT 100MHz fast speed @ 1.8V pulldown"
io8_100m_ft_ms_1v8  "IO8_FT 100MHz med speed @ 1.8V"
io8_100m_ft_ms_pu_1v8  "IO8_FT 100MHz med speed @ 1.8V pullup"
io8_100m_ft_ms_pd_1v8  "IO8_FT 100MHz med speed @ 1.8V pulldown"
io8_100m_ft_ls_1v8  "IO8_FT 100MHz low speed @ 1.8V"
io8_100m_ft_ls_pu_1v8  "IO8_FT 100MHz low speed @ 1.8V pullup"
io8_100m_ft_ls_pd_1v8  "IO8_FT 100MHz low speed @ 1.8V pulldown"
io8_100m_ft_hs_3v3  "IO8_FT 100MHz high speed @ 3.3V"
io8_100m_ft_hs_pu_3v3  "IO8_FT 100MHz high speed @ 3.3V pullup"
io8_100m_ft_hs_pd_3v3  "IO8_FT 100MHz high speed @ 3.3V pulldown"
io8_100m_ft_fs_3v3  "IO8_FT 100MHz fast speed @ 3.3V"
io8_100m_ft_fs_pu_3v3  "IO8_FT 100MHz fast speed @ 3.3V pullup"
io8_100m_ft_fs_pd_3v3  "IO8_FT 100MHz fast speed @ 3.3V pulldown"
io8_100m_ft_ms_3v3  "IO8_FT 100MHz med speed @ 3.3V"
io8_100m_ft_ms_pu_3v3  "IO8_FT 100MHz med speed @ 3.3V pullup"
io8_100m_ft_ms_pd_3v3  "IO8_FT 100MHz med speed @ 3.3V pulldown"
io8_100m_ft_ls_3v3  "IO8_FT 100MHz low speed @ 3.3V"
io8_100m_ft_ls_pu_3v3  "IO8_FT 100MHz low speed @ 3.3V pullup"
io8_100m_ft_ls_pd_3v3  "IO8_FT 100MHz low speed @ 3.3V pulldown"
io8_ft_v33_hs_1v2  "IO8_FT_V33 high speed @ 1.2V"
io8_ft_v33_hs_pu_1v2  "IO8_FT_V33 high speed @ 1.2V pullup"
io8_ft_v33_hs_pd_1v2  "IO8_FT_V33 high speed @ 1.2V pulldown"
io8_ft_v33_fs_1v2  "IO8_FT_V33 fast speed @ 1.2V"
io8_ft_v33_fs_pu_1v2  "IO8_FT_V33 fast speed @ 1.2V pullup"
io8_ft_v33_fs_pd_1v2  "IO8_FT_V33 fast speed @ 1.2V pulldown"
io8_ft_v33_ms_1v2  "IO8_FT_V33 med speed @ 1.2V"
io8_ft_v33_ms_pu_1v2  "IO8_FT_V33 med speed @ 1.2V pullup"
io8_ft_v33_ms_pd_1v2  "IO8_FT_V33 med speed @ 1.2V pulldown"
io8_ft_v33_ls_1v2  "IO8_FT_V33 low speed @ 1.2V"
io8_ft_v33_ls_pu_1v2  "IO8_FT_V33 low speed @ 1.2V pullup"
io8_ft_v33_ls_pd_1v2  "IO8_FT_V33 low speed @ 1.2V pulldown"
io8_ft_v33_hs_1v8  "IO8_FT_V33 high speed @ 1.8V"
io8_ft_v33_hs_pu_1v8  "IO8_FT_V33 high speed @ 1.8V pullup"
io8_ft_v33_hs_pd_1v8  "IO8_FT_V33 high speed @ 1.8V pulldown"
io8_ft_v33_fs_1v8  "IO8_FT_V33 fast speed @ 1.8V"
io8_ft_v33_fs_pu_1v8  "IO8_FT_V33 fast speed @ 1.8V pullup"
io8_ft_v33_fs_pd_1v8  "IO8_FT_V33 fast speed @ 1.8V pulldown"
io8_ft_v33_ms_1v8  "IO8_FT_V33 med speed @ 1.8V"
io8_ft_v33_ms_pu_1v8  "IO8_FT_V33 med speed @ 1.8V pullup"
io8_ft_v33_ms_pd_1v8  "IO8_FT_V33 med speed @ 1.8V pulldown"
io8_ft_v33_ls_1v8  "IO8_FT_V33 low speed @ 1.8V"
io8_ft_v33_ls_pu_1v8  "IO8_FT_V33 low speed @ 1.8V pullup"
io8_ft_v33_ls_pd_1v8  "IO8_FT_V33 low speed @ 1.8V pulldown"
io8_ft_v33_hs_3v3  "IO8_FT_V33 high speed @ 3.3V"
io8_ft_v33_hs_pu_3v3  "IO8_FT_V33 high speed @ 3.3V pullup"
io8_ft_v33_hs_pd_3v3  "IO8_FT_V33 high speed @ 3.3V pulldown"
io8_ft_v33_fs_3v3  "IO8_FT_V33 fast speed @ 3.3V"
io8_ft_v33_fs_pu_3v3  "IO8_FT_V33 fast speed @ 3.3V pullup"
io8_ft_v33_fs_pd_3v3  "IO8_FT_V33 fast speed @ 3.3V pulldown"
io8_ft_v33_ms_3v3  "IO8_FT_V33 med speed @ 3.3V"
io8_ft_v33_ms_pu_3v3  "IO8_FT_V33 med speed @ 3.3V pullup"
io8_ft_v33_ms_pd_3v3  "IO8_FT_V33 med speed @ 3.3V pulldown"
io8_ft_v33_ls_3v3  "IO8_FT_V33 low speed @ 3.3V"
io8_ft_v33_ls_pu_3v3  "IO8_FT_V33 low speed @ 3.3V pullup"
io8_ft_v33_ls_pd_3v3  "IO8_FT_V33 low speed @ 3.3V pulldown"
[Model Selector] io8_usb_ft
io8_100m_ft_hs_1v2  "IO8_FT 100MHz high speed @ 1.2V"
io8_100m_ft_hs_pu_1v2  "IO8_FT 100MHz high speed @ 1.2V pullup"
io8_100m_ft_hs_pd_1v2  "IO8_FT 100MHz high speed @ 1.2V pulldown"
io8_100m_ft_fs_1v2  "IO8_FT 100MHz fast speed @ 1.2V"
io8_100m_ft_fs_pu_1v2  "IO8_FT 100MHz fast speed @ 1.2V pullup"
io8_100m_ft_fs_pd_1v2  "IO8_FT 100MHz fast speed @ 1.2V pulldown"
io8_100m_ft_ms_1v2  "IO8_FT 100MHz med speed @ 1.2V"
io8_100m_ft_ms_pu_1v2  "IO8_FT 100MHz med speed @ 1.2V pullup"
io8_100m_ft_ms_pd_1v2  "IO8_FT 100MHz med speed @ 1.2V pulldown"
io8_100m_ft_ls_1v2  "IO8_FT 100MHz low speed @ 1.2V"
io8_100m_ft_ls_pu_1v2  "IO8_FT 100MHz low speed @ 1.2V pullup"
io8_100m_ft_ls_pd_1v2  "IO8_FT 100MHz low speed @ 1.2V pulldown"
io8_100m_ft_hs_1v8  "IO8_FT 100MHz high speed @ 1.8V"
io8_100m_ft_hs_pu_1v8  "IO8_FT 100MHz high speed @ 1.8V pullup"
io8_100m_ft_hs_pd_1v8  "IO8_FT 100MHz high speed @ 1.8V pulldown"
io8_100m_ft_fs_1v8  "IO8_FT 100MHz fast speed @ 1.8V"
io8_100m_ft_fs_pu_1v8  "IO8_FT 100MHz fast speed @ 1.8V pullup"
io8_100m_ft_fs_pd_1v8  "IO8_FT 100MHz fast speed @ 1.8V pulldown"
io8_100m_ft_ms_1v8  "IO8_FT 100MHz med speed @ 1.8V"
io8_100m_ft_ms_pu_1v8  "IO8_FT 100MHz med speed @ 1.8V pullup"
io8_100m_ft_ms_pd_1v8  "IO8_FT 100MHz med speed @ 1.8V pulldown"
io8_100m_ft_ls_1v8  "IO8_FT 100MHz low speed @ 1.8V"
io8_100m_ft_ls_pu_1v8  "IO8_FT 100MHz low speed @ 1.8V pullup"
io8_100m_ft_ls_pd_1v8  "IO8_FT 100MHz low speed @ 1.8V pulldown"
io8_100m_ft_hs_3v3  "IO8_FT 100MHz high speed @ 3.3V"
io8_100m_ft_hs_pu_3v3  "IO8_FT 100MHz high speed @ 3.3V pullup"
io8_100m_ft_hs_pd_3v3  "IO8_FT 100MHz high speed @ 3.3V pulldown"
io8_100m_ft_fs_3v3  "IO8_FT 100MHz fast speed @ 3.3V"
io8_100m_ft_fs_pu_3v3  "IO8_FT 100MHz fast speed @ 3.3V pullup"
io8_100m_ft_fs_pd_3v3  "IO8_FT 100MHz fast speed @ 3.3V pulldown"
io8_100m_ft_ms_3v3  "IO8_FT 100MHz med speed @ 3.3V"
io8_100m_ft_ms_pu_3v3  "IO8_FT 100MHz med speed @ 3.3V pullup"
io8_100m_ft_ms_pd_3v3  "IO8_FT 100MHz med speed @ 3.3V pulldown"
io8_100m_ft_ls_3v3  "IO8_FT 100MHz low speed @ 3.3V"
io8_100m_ft_ls_pu_3v3  "IO8_FT 100MHz low speed @ 3.3V pullup"
io8_100m_ft_ls_pd_3v3  "IO8_FT 100MHz low speed @ 3.3V pulldown"
io8_usb_fs_3v3  "IOUSB fast speed @ 3.3V"
io8_usb_fs_pu1_3v3  "IO8USB fast speed @ 3.3V pullup1"
io8_usb_fs_pd1_3v3  "IOUSB fast speed @ 3.3V pulldown1"
io8_usb_ls_3v3  "IOUSB low speed @ 3.3V"
io8_usb_ls_pu1_3v3  "IOUSB low speed @ 3.3V pullup1"
io8_usb_ls_pd1_3v3  "IOUSB low speed @ 3.3V pulldown1"
io8_usb_fs_pu2_3v3  "IOUSB fast speed @ 3.3V pullup2"
io8_usb_fs_pd2_3v3  "IOUSB fast speed @ 3.3V pulldown2"
io8_usb_ls_pu2_3v3  "IOUSB low speed @ 3.3V pullup2"
io8_usb_ls_pd2_3v3  "IOUSB low speed @ 3.3V pulldown2"
[Model Selector] io8_166m_hslv_ft
io8_166m_ft_hs_1v2  "IO8_FT 166MHz high speed @ 1.2V"
io8_166m_ft_hs_pu_1v2  "IO8_FT 166MHz high speed @ 1.2V pullup"
io8_166m_ft_hs_pd_1v2  "IO8_FT 166MHz high speed @ 1.2V pulldown"
io8_166m_ft_fs_1v2  "IO8_FT 166MHz fast speed @ 1.2V"
io8_166m_ft_fs_pu_1v2  "IO8_FT 166MHz fast speed @ 1.2V pullup"
io8_166m_ft_fs_pd_1v2  "IO8_FT 166MHz fast speed @ 1.2V pulldown"
io8_166m_ft_ms_1v2  "IO8_FT 166MHz med speed @ 1.2V"
io8_166m_ft_ms_pu_1v2  "IO8_FT 166MHz med speed @ 1.2V pullup"
io8_166m_ft_ms_pd_1v2  "IO8_FT 166MHz med speed @ 1.2V pulldown"
io8_166m_ft_ls_1v2  "IO8_FT 166MHz low speed @ 1.2V"
io8_166m_ft_ls_pu_1v2  "IO8_FT 166MHz low speed @ 1.2V pullup"
io8_166m_ft_ls_pd_1v2  "IO8_FT 166MHz low speed @ 1.2V pulldown"
io8_166m_ft_hs_1v8  "IO8_FT 166MHz high speed @ 1.8V"
io8_166m_ft_hs_pu_1v8  "IO8_FT 166MHz high speed @ 1.8V pullup"
io8_166m_ft_hs_pd_1v8  "IO8_FT 166MHz high speed @ 1.8V pulldown"
io8_166m_ft_fs_1v8  "IO8_FT 166MHz fast speed @ 1.8V"
io8_166m_ft_fs_pu_1v8  "IO8_FT 166MHz fast speed @ 1.8V pullup"
io8_166m_ft_fs_pd_1v8  "IO8_FT 166MHz fast speed @ 1.8V pulldown"
io8_166m_ft_ms_1v8  "IO8_FT 166MHz med speed @ 1.8V"
io8_166m_ft_ms_pu_1v8  "IO8_FT 166MHz med speed @ 1.8V pullup"
io8_166m_ft_ms_pd_1v8  "IO8_FT 166MHz med speed @ 1.8V pulldown"
io8_166m_ft_ls_1v8  "IO8_FT 166MHz low speed @ 1.8V"
io8_166m_ft_ls_pu_1v8  "IO8_FT 166MHz low speed @ 1.8V pullup"
io8_166m_ft_ls_pd_1v8  "IO8_FT 166MHz low speed @ 1.8V pulldown"
io8_166m_ft_hs_3v3  "IO8_FT 166MHz high speed @ 3.3V"
io8_166m_ft_hs_pu_3v3  "IO8_FT 166MHz high speed @ 3.3V pullup"
io8_166m_ft_hs_pd_3v3  "IO8_FT 166MHz high speed @ 3.3V pulldown"
io8_166m_ft_fs_3v3  "IO8_FT 166MHz fast speed @ 3.3V"
io8_166m_ft_fs_pu_3v3  "IO8_FT 166MHz fast speed @ 3.3V pullup"
io8_166m_ft_fs_pd_3v3  "IO8_FT 166MHz fast speed @ 3.3V pulldown"
io8_166m_ft_ms_3v3  "IO8_FT 166MHz med speed @ 3.3V"
io8_166m_ft_ms_pu_3v3  "IO8_FT 166MHz med speed @ 3.3V pullup"
io8_166m_ft_ms_pd_3v3  "IO8_FT 166MHz med speed @ 3.3V pulldown"
io8_166m_ft_ls_3v3  "IO8_FT 166MHz low speed @ 3.3V"
io8_166m_ft_ls_pu_3v3  "IO8_FT 166MHz low speed @ 3.3V pullup"
io8_166m_ft_ls_pd_3v3  "IO8_FT 166MHz low speed @ 3.3V pulldown"
io8_166m_hslv_ft_hs_1v2  "IO8_FT 166MHz HSLV high speed @ 1.2V"
io8_166m_hslv_ft_hs_pu_1v2  "IO8_FT 166MHz HSLV high speed @ 1.2V pullup"
io8_166m_hslv_ft_hs_pd_1v2  "IO8_FT 166MHz HSLV high speed @ 1.2V pulldown"
io8_166m_hslv_ft_fs_1v2  "IO8_FT 166MHz HSLV fast speed @ 1.2V"
io8_166m_hslv_ft_fs_pu_1v2  "IO8_FT 166MHz HSLV fast speed @ 1.2V pullup"
io8_166m_hslv_ft_fs_pd_1v2  "IO8_FT 166MHz HSLV fast speed @ 1.2V pulldown"
io8_166m_hslv_ft_ms_1v2  "IO8_FT 166MHz HSLV med speed @ 1.2V"
io8_166m_hslv_ft_ms_pu_1v2  "IO8_FT 166MHz HSLV med speed @ 1.2V pullup"
io8_166m_hslv_ft_ms_pd_1v2  "IO8_FT 166MHz HSLV med speed @ 1.2V pulldown"
io8_166m_hslv_ft_ls_1v2  "IO8_FT 166MHz HSLV low speed @ 1.2V"
io8_166m_hslv_ft_ls_pu_1v2  "IO8_FT 166MHz HSLV low speed @ 1.2V pullup"
io8_166m_hslv_ft_ls_pd_1v2  "IO8_FT 166MHz HSLV low speed @ 1.2V pulldown"
io8_166m_hslv_ft_hs_1v8  "IO8_FT 166MHz HSLV high speed @ 1.8V"
io8_166m_hslv_ft_hs_pu_1v8  "IO8_FT 166MHz HSLV high speed @ 1.8V pullup"
io8_166m_hslv_ft_hs_pd_1v8  "IO8_FT 166MHz HSLV high speed @ 1.8V pulldown"
io8_166m_hslv_ft_fs_1v8  "IO8_FT 166MHz HSLV fast speed @ 1.8V"
io8_166m_hslv_ft_fs_pu_1v8  "IO8_FT 166MHz HSLV fast speed @ 1.8V pullup"
io8_166m_hslv_ft_fs_pd_1v8  "IO8_FT 166MHz HSLV fast speed @ 1.8V pulldown"
io8_166m_hslv_ft_ms_1v8  "IO8_FT 166MHz HSLV med speed @ 1.8V"
io8_166m_hslv_ft_ms_pu_1v8  "IO8_FT 166MHz HSLV med speed @ 1.8V pullup"
io8_166m_hslv_ft_ms_pd_1v8  "IO8_FT 166MHz HSLV med speed @ 1.8V pulldown"
io8_166m_hslv_ft_ls_1v8  "IO8_FT 166MHz HSLV low speed @ 1.8V"
io8_166m_hslv_ft_ls_pu_1v8  "IO8_FT 166MHz HSLV low speed @ 1.8V pullup"
io8_166m_hslv_ft_ls_pd_1v8  "IO8_FT 166MHz HSLV low speed @ 1.8V pulldown"
io8_166m_hslv_ft_hs_2v5  "IO8_FT 166MHz HSLV high speed @ 2.5V"
io8_166m_hslv_ft_hs_pu_2v5  "IO8_FT 166MHz HSLV high speed @ 2.5V pullup"
io8_166m_hslv_ft_hs_pd_2v5  "IO8_FT 166MHz HSLV high speed @ 2.5V pulldown"
io8_166m_hslv_ft_fs_2v5  "IO8_FT 166MHz HSLV fast speed @ 2.5V"
io8_166m_hslv_ft_fs_pu_2v5  "IO8_FT 166MHz HSLV fast speed @ 2.5V pullup"
io8_166m_hslv_ft_fs_pd_2v5  "IO8_FT 166MHz HSLV fast speed @ 2.5V pulldown"
io8_166m_hslv_ft_ms_2v5  "IO8_FT 166MHz HSLV med speed @ 2.5V"
io8_166m_hslv_ft_ms_pu_2v5  "IO8_FT 166MHz HSLV med speed @ 2.5V pullup"
io8_166m_hslv_ft_ms_pd_2v5  "IO8_FT 166MHz HSLV med speed @ 2.5V pulldown"
io8_166m_hslv_ft_ls_2v5  "IO8_FT 166MHz HSLV low speed @ 2.5V"
io8_166m_hslv_ft_ls_pu_2v5  "IO8_FT 166MHz HSLV low speed @ 2.5V pullup"
io8_166m_hslv_ft_ls_pd_2v5  "IO8_FT 166MHz HSLV low speed @ 2.5V pulldown"
[Model Selector] io8_166m_hslv_i2c_ft
io8_166m_ft_hs_1v2  "IO8_FT 166MHz high speed @ 1.2V"
io8_166m_ft_hs_pu_1v2  "IO8_FT 166MHz high speed @ 1.2V pullup"
io8_166m_ft_hs_pd_1v2  "IO8_FT 166MHz high speed @ 1.2V pulldown"
io8_166m_ft_fs_1v2  "IO8_FT 166MHz fast speed @ 1.2V"
io8_166m_ft_fs_pu_1v2  "IO8_FT 166MHz fast speed @ 1.2V pullup"
io8_166m_ft_fs_pd_1v2  "IO8_FT 166MHz fast speed @ 1.2V pulldown"
io8_166m_ft_ms_1v2  "IO8_FT 166MHz med speed @ 1.2V"
io8_166m_ft_ms_pu_1v2  "IO8_FT 166MHz med speed @ 1.2V pullup"
io8_166m_ft_ms_pd_1v2  "IO8_FT 166MHz med speed @ 1.2V pulldown"
io8_166m_ft_ls_1v2  "IO8_FT 166MHz low speed @ 1.2V"
io8_166m_ft_ls_pu_1v2  "IO8_FT 166MHz low speed @ 1.2V pullup"
io8_166m_ft_ls_pd_1v2  "IO8_FT 166MHz low speed @ 1.2V pulldown"
io8_166m_ft_hs_1v8  "IO8_FT 166MHz high speed @ 1.8V"
io8_166m_ft_hs_pu_1v8  "IO8_FT 166MHz high speed @ 1.8V pullup"
io8_166m_ft_hs_pd_1v8  "IO8_FT 166MHz high speed @ 1.8V pulldown"
io8_166m_ft_fs_1v8  "IO8_FT 166MHz fast speed @ 1.8V"
io8_166m_ft_fs_pu_1v8  "IO8_FT 166MHz fast speed @ 1.8V pullup"
io8_166m_ft_fs_pd_1v8  "IO8_FT 166MHz fast speed @ 1.8V pulldown"
io8_166m_ft_ms_1v8  "IO8_FT 166MHz med speed @ 1.8V"
io8_166m_ft_ms_pu_1v8  "IO8_FT 166MHz med speed @ 1.8V pullup"
io8_166m_ft_ms_pd_1v8  "IO8_FT 166MHz med speed @ 1.8V pulldown"
io8_166m_ft_ls_1v8  "IO8_FT 166MHz low speed @ 1.8V"
io8_166m_ft_ls_pu_1v8  "IO8_FT 166MHz low speed @ 1.8V pullup"
io8_166m_ft_ls_pd_1v8  "IO8_FT 166MHz low speed @ 1.8V pulldown"
io8_166m_ft_hs_3v3  "IO8_FT 166MHz high speed @ 3.3V"
io8_166m_ft_hs_pu_3v3  "IO8_FT 166MHz high speed @ 3.3V pullup"
io8_166m_ft_hs_pd_3v3  "IO8_FT 166MHz high speed @ 3.3V pulldown"
io8_166m_ft_fs_3v3  "IO8_FT 166MHz fast speed @ 3.3V"
io8_166m_ft_fs_pu_3v3  "IO8_FT 166MHz fast speed @ 3.3V pullup"
io8_166m_ft_fs_pd_3v3  "IO8_FT 166MHz fast speed @ 3.3V pulldown"
io8_166m_ft_ms_3v3  "IO8_FT 166MHz med speed @ 3.3V"
io8_166m_ft_ms_pu_3v3  "IO8_FT 166MHz med speed @ 3.3V pullup"
io8_166m_ft_ms_pd_3v3  "IO8_FT 166MHz med speed @ 3.3V pulldown"
io8_166m_ft_ls_3v3  "IO8_FT 166MHz low speed @ 3.3V"
io8_166m_ft_ls_pu_3v3  "IO8_FT 166MHz low speed @ 3.3V pullup"
io8_166m_ft_ls_pd_3v3  "IO8_FT 166MHz low speed @ 3.3V pulldown"
io8_166m_hslv_ft_hs_1v2  "IO8_FT 166MHz HSLV high speed @ 1.2V"
io8_166m_hslv_ft_hs_pu_1v2  "IO8_FT 166MHz HSLV high speed @ 1.2V pullup"
io8_166m_hslv_ft_hs_pd_1v2  "IO8_FT 166MHz HSLV high speed @ 1.2V pulldown"
io8_166m_hslv_ft_fs_1v2  "IO8_FT 166MHz HSLV fast speed @ 1.2V"
io8_166m_hslv_ft_fs_pu_1v2  "IO8_FT 166MHz HSLV fast speed @ 1.2V pullup"
io8_166m_hslv_ft_fs_pd_1v2  "IO8_FT 166MHz HSLV fast speed @ 1.2V pulldown"
io8_166m_hslv_ft_ms_1v2  "IO8_FT 166MHz HSLV med speed @ 1.2V"
io8_166m_hslv_ft_ms_pu_1v2  "IO8_FT 166MHz HSLV med speed @ 1.2V pullup"
io8_166m_hslv_ft_ms_pd_1v2  "IO8_FT 166MHz HSLV med speed @ 1.2V pulldown"
io8_166m_hslv_ft_ls_1v2  "IO8_FT 166MHz HSLV low speed @ 1.2V"
io8_166m_hslv_ft_ls_pu_1v2  "IO8_FT 166MHz HSLV low speed @ 1.2V pullup"
io8_166m_hslv_ft_ls_pd_1v2  "IO8_FT 166MHz HSLV low speed @ 1.2V pulldown"
io8_166m_hslv_ft_hs_1v8  "IO8_FT 166MHz HSLV high speed @ 1.8V"
io8_166m_hslv_ft_hs_pu_1v8  "IO8_FT 166MHz HSLV high speed @ 1.8V pullup"
io8_166m_hslv_ft_hs_pd_1v8  "IO8_FT 166MHz HSLV high speed @ 1.8V pulldown"
io8_166m_hslv_ft_fs_1v8  "IO8_FT 166MHz HSLV fast speed @ 1.8V"
io8_166m_hslv_ft_fs_pu_1v8  "IO8_FT 166MHz HSLV fast speed @ 1.8V pullup"
io8_166m_hslv_ft_fs_pd_1v8  "IO8_FT 166MHz HSLV fast speed @ 1.8V pulldown"
io8_166m_hslv_ft_ms_1v8  "IO8_FT 166MHz HSLV med speed @ 1.8V"
io8_166m_hslv_ft_ms_pu_1v8  "IO8_FT 166MHz HSLV med speed @ 1.8V pullup"
io8_166m_hslv_ft_ms_pd_1v8  "IO8_FT 166MHz HSLV med speed @ 1.8V pulldown"
io8_166m_hslv_ft_ls_1v8  "IO8_FT 166MHz HSLV low speed @ 1.8V"
io8_166m_hslv_ft_ls_pu_1v8  "IO8_FT 166MHz HSLV low speed @ 1.8V pullup"
io8_166m_hslv_ft_ls_pd_1v8  "IO8_FT 166MHz HSLV low speed @ 1.8V pulldown"
io8_166m_hslv_ft_hs_2v5  "IO8_FT 166MHz HSLV high speed @ 2.5V"
io8_166m_hslv_ft_hs_pu_2v5  "IO8_FT 166MHz HSLV high speed @ 2.5V pullup"
io8_166m_hslv_ft_hs_pd_2v5  "IO8_FT 166MHz HSLV high speed @ 2.5V pulldown"
io8_166m_hslv_ft_fs_2v5  "IO8_FT 166MHz HSLV fast speed @ 2.5V"
io8_166m_hslv_ft_fs_pu_2v5  "IO8_FT 166MHz HSLV fast speed @ 2.5V pullup"
io8_166m_hslv_ft_fs_pd_2v5  "IO8_FT 166MHz HSLV fast speed @ 2.5V pulldown"
io8_166m_hslv_ft_ms_2v5  "IO8_FT 166MHz HSLV med speed @ 2.5V"
io8_166m_hslv_ft_ms_pu_2v5  "IO8_FT 166MHz HSLV med speed @ 2.5V pullup"
io8_166m_hslv_ft_ms_pd_2v5  "IO8_FT 166MHz HSLV med speed @ 2.5V pulldown"
io8_166m_hslv_ft_ls_2v5  "IO8_FT 166MHz HSLV low speed @ 2.5V"
io8_166m_hslv_ft_ls_pu_2v5  "IO8_FT 166MHz HSLV low speed @ 2.5V pullup"
io8_166m_hslv_ft_ls_pd_2v5  "IO8_FT 166MHz HSLV low speed @ 2.5V pulldown"
io8_166m_i2c_ft_1v2  "IO8_FT 166MHz I2C @ 1.2V"
io8_166m_i2c_ft_pu_1v2  "IO8_FT 166MHz I2C @ 1.2V pullup"
io8_166m_i2c_ft_pd_1v2  "IO8_FT 166MHz I2C @ 1.2V pulldown"
io8_166m_i2c_ft_1v8  "IO8_FT 166MHz I2C @ 1.8V"
io8_166m_i2c_ft_pu_1v8  "IO8_FT 166MHz I2C @ 1.8V pullup"
io8_166m_i2c_ft_pd_1v8  "IO8_FT 166MHz I2C @ 1,8V pulldown"
io8_166m_i2c_ft_3v3  "IO8_FT 166MHz I2C @ 3.3V"
io8_166m_i2c_ft_pu_3v3  "IO8_FT 166MHz I2C HSLV @ 3.3V pullup"
io8_166m_i2c_ft_pd_3v3  "IO8_FT 166MHz I2C @ 3.3V pulldown"
[Model Selector] io8_100m_ft_v33
io8_ft_v33_hs_1v2  "IO8_FT_V33 high speed @ 1.2V"
io8_ft_v33_hs_pu_1v2  "IO8_FT_V33 high speed @ 1.2V pullup"
io8_ft_v33_hs_pd_1v2  "IO8_FT_V33 high speed @ 1.2V pulldown"
io8_ft_v33_fs_1v2  "IO8_FT_V33 fast speed @ 1.2V"
io8_ft_v33_fs_pu_1v2  "IO8_FT_V33 fast speed @ 1.2V pullup"
io8_ft_v33_fs_pd_1v2  "IO8_FT_V33 fast speed @ 1.2V pulldown"
io8_ft_v33_ms_1v2  "IO8_FT_V33 med speed @ 1.2V"
io8_ft_v33_ms_pu_1v2  "IO8_FT_V33 med speed @ 1.2V pullup"
io8_ft_v33_ms_pd_1v2  "IO8_FT_V33 med speed @ 1.2V pulldown"
io8_ft_v33_ls_1v2  "IO8_FT_V33 low speed @ 1.2V"
io8_ft_v33_ls_pu_1v2  "IO8_FT_V33 low speed @ 1.2V pullup"
io8_ft_v33_ls_pd_1v2  "IO8_FT_V33 low speed @ 1.2V pulldown"
io8_ft_v33_hs_1v8  "IO8_FT_V33 high speed @ 1.8V"
io8_ft_v33_hs_pu_1v8  "IO8_FT_V33 high speed @ 1.8V pullup"
io8_ft_v33_hs_pd_1v8  "IO8_FT_V33 high speed @ 1.8V pulldown"
io8_ft_v33_fs_1v8  "IO8_FT_V33 fast speed @ 1.8V"
io8_ft_v33_fs_pu_1v8  "IO8_FT_V33 fast speed @ 1.8V pullup"
io8_ft_v33_fs_pd_1v8  "IO8_FT_V33 fast speed @ 1.8V pulldown"
io8_ft_v33_ms_1v8  "IO8_FT_V33 med speed @ 1.8V"
io8_ft_v33_ms_pu_1v8  "IO8_FT_V33 med speed @ 1.8V pullup"
io8_ft_v33_ms_pd_1v8  "IO8_FT_V33 med speed @ 1.8V pulldown"
io8_ft_v33_ls_1v8  "IO8_FT_V33 low speed @ 1.8V"
io8_ft_v33_ls_pu_1v8  "IO8_FT_V33 low speed @ 1.8V pullup"
io8_ft_v33_ls_pd_1v8  "IO8_FT_V33 low speed @ 1.8V pulldown"
io8_ft_v33_hs_3v3  "IO8_FT_V33 high speed @ 3.3V"
io8_ft_v33_hs_pu_3v3  "IO8_FT_V33 high speed @ 3.3V pullup"
io8_ft_v33_hs_pd_3v3  "IO8_FT_V33 high speed @ 3.3V pulldown"
io8_ft_v33_fs_3v3  "IO8_FT_V33 fast speed @ 3.3V"
io8_ft_v33_fs_pu_3v3  "IO8_FT_V33 fast speed @ 3.3V pullup"
io8_ft_v33_fs_pd_3v3  "IO8_FT_V33 fast speed @ 3.3V pulldown"
io8_ft_v33_ms_3v3  "IO8_FT_V33 med speed @ 3.3V"
io8_ft_v33_ms_pu_3v3  "IO8_FT_V33 med speed @ 3.3V pullup"
io8_ft_v33_ms_pd_3v3  "IO8_FT_V33 med speed @ 3.3V pulldown"
io8_ft_v33_ls_3v3  "IO8_FT_V33 low speed @ 3.3V"
io8_ft_v33_ls_pu_3v3  "IO8_FT_V33 low speed @ 3.3V pullup"
io8_ft_v33_ls_pd_3v3  "IO8_FT_V33 low speed @ 3.3V pulldown"
[Define Package Model]  455-ufbga-7x7-100-ldo-100mhz-230421
[Manufacturer]  unknown
[OEM]  unknown
[Description]  unknown
[Number Of Pins]  92
[Pin Numbers]
| Pin Name Terminal   Net Name   Starting Node   Ending Node
H2 | NRST
L2 | PA0
M2 | PA1
K3 | PA2
L3 | PA3
M3 | PA4
K4 | PA5
L4 | PA6
M4 | PA7
D11 | PA8
D10 | PA9
C12 | PA10
B12 | PA11
A12 | PA12
A11 | PA13
A10 | PA14
A9 | PA15
M5 | PB0
M6 | PB1
L6 | PB2
A8 | PB3
A7 | PB4
C5 | PB5
B5 | PB6
B4 | PB7
A3 | PB8
B3 | PB9
L10 | PB10
L12 | PB12
K12 | PB13
K11 | PB14
K10 | PB15
H1 | PC0
J2 | PC1
J3 | PC2
K2 | PC3
K5 | PC4
L5 | PC5
E12 | PC6
E11 | PC7
E10 | PC8
D12 | PC9
B11 | PC10
C10 | PC11
B10 | PC12
C1 | PC13
D1 | PC14-OSC32_IN
E1 | PC15-OSC32_OUT
C9 | PD0
B9 | PD1
C8 | PD2
B8 | PD3
B7 | PD4
A6 | PD5
B6 | PD6
A5 | PD7
K9 | PD8
K8 | PD9
J12 | PD10
J11 | PD11
J10 | PD12
H12 | PD13
H11 | PD14
H10 | PD15
C3 | PE0
A2 | PE1
B2 | PE2
A1 | PE3
B1 | PE4
C2 | PE5
D2 | PE6
M7 | PE7
L7 | PE8
M8 | PE9
L8 | PE10
M9 | PE11
L9 | PE12
M10 | PE13
M11 | PE14
M12 | PE15
F1 | PH0-OSC_IN
G1 | PH1-OSC_OUT
A4 | PH3-BOOT0
E2 | VBAT
L11 | VCAP
C4 | VDD
M1 | VDDA
C11 | VDDUSB
K1 | VREFM
L1 | VREFP
D3 | VSS
J1 | VSSA
|[Merged Pins]  D3
|E3  |  VSS
|F2  |  VSS
|F11  |  VSS
|F12  |  VSS
|[Merged Pins]  C4
|G2  |  VDD
|G11  |  VDD
|G12  |  VDD
|H3  |  VDD
[Model Data]
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[End Model Data]
[End Package Model]
| Models and submodels in the file (208): io8_100m_ft_hs_1v2 (I/O), io8_100m_ft_hs_pu_1v2 (I/O), io8_100m_ft_hs_pd_1v2 (I/O), io8_100m_ft_fs_1v2 (I/O), io8_100m_ft_fs_pu_1v2 (I/O), io8_100m_ft_fs_pd_1v2 (I/O), io8_100m_ft_ms_1v2 (I/O), io8_100m_ft_ms_pu_1v2 (I/O), io8_100m_ft_ms_pd_1v2 (I/O), io8_100m_ft_ls_1v2 (I/O), io8_100m_ft_ls_pu_1v2 (I/O), io8_100m_ft_ls_pd_1v2 (I/O), io8_100m_ft_hs_1v8 (I/O), io8_100m_ft_hs_pu_1v8 (I/O), io8_100m_ft_hs_pd_1v8 (I/O), io8_100m_ft_fs_1v8 (I/O), io8_100m_ft_fs_pu_1v8 (I/O), io8_100m_ft_fs_pd_1v8 (I/O), io8_100m_ft_ms_1v8 (I/O), io8_100m_ft_ms_pu_1v8 (I/O), io8_100m_ft_ms_pd_1v8 (I/O), io8_100m_ft_ls_1v8 (I/O), io8_100m_ft_ls_pu_1v8 (I/O), io8_100m_ft_ls_pd_1v8 (I/O), io8_100m_ft_hs_3v3 (I/O), io8_100m_ft_hs_pu_3v3 (I/O), io8_100m_ft_hs_pd_3v3 (I/O), io8_100m_ft_fs_3v3 (I/O), io8_100m_ft_fs_pu_3v3 (I/O), io8_100m_ft_fs_pd_3v3 (I/O), io8_100m_ft_ms_3v3 (I/O), io8_100m_ft_ms_pu_3v3 (I/O), io8_100m_ft_ms_pd_3v3 (I/O), io8_100m_ft_ls_3v3 (I/O), io8_100m_ft_ls_pu_3v3 (I/O), io8_100m_ft_ls_pd_3v3 (I/O), io8_100m_hslv_ft_hs_1v2 (I/O), io8_100m_hslv_ft_hs_pu_1v2 (I/O), io8_100m_hslv_ft_hs_pd_1v2 (I/O), io8_100m_hslv_ft_fs_1v2 (I/O), io8_100m_hslv_ft_fs_pu_1v2 (I/O), io8_100m_hslv_ft_fs_pd_1v2 (I/O), io8_100m_hslv_ft_ms_1v2 (I/O), io8_100m_hslv_ft_ms_pu_1v2 (I/O), io8_100m_hslv_ft_ms_pd_1v2 (I/O), io8_100m_hslv_ft_ls_1v2 (I/O), io8_100m_hslv_ft_ls_pu_1v2 (I/O), io8_100m_hslv_ft_ls_pd_1v2 (I/O), io8_100m_hslv_ft_hs_1v8 (I/O), io8_100m_hslv_ft_hs_pu_1v8 (I/O), io8_100m_hslv_ft_hs_pd_1v8 (I/O), io8_100m_hslv_ft_fs_1v8 (I/O), io8_100m_hslv_ft_fs_pu_1v8 (I/O), io8_100m_hslv_ft_fs_pd_1v8 (I/O), io8_100m_hslv_ft_ms_1v8 (I/O), io8_100m_hslv_ft_ms_pu_1v8 (I/O), io8_100m_hslv_ft_ms_pd_1v8 (I/O), io8_100m_hslv_ft_ls_1v8 (I/O), io8_100m_hslv_ft_ls_pu_1v8 (I/O), io8_100m_hslv_ft_ls_pd_1v8 (I/O), io8_100m_hslv_ft_hs_2v5 (I/O), io8_100m_hslv_ft_hs_pu_2v5 (I/O), io8_100m_hslv_ft_hs_pd_2v5 (I/O), io8_100m_hslv_ft_fs_2v5 (I/O), io8_100m_hslv_ft_fs_pu_2v5 (I/O), io8_100m_hslv_ft_fs_pd_2v5 (I/O), io8_100m_hslv_ft_ms_2v5 (I/O), io8_100m_hslv_ft_ms_pu_2v5 (I/O), io8_100m_hslv_ft_ms_pd_2v5 (I/O), io8_100m_hslv_ft_ls_2v5 (I/O), io8_100m_hslv_ft_ls_pu_2v5 (I/O), io8_100m_hslv_ft_ls_pd_2v5 (I/O), io8_166m_ft_hs_1v2 (I/O), io8_166m_ft_hs_pu_1v2 (I/O), io8_166m_ft_hs_pd_1v2 (I/O), io8_166m_ft_fs_1v2 (I/O), io8_166m_ft_fs_pu_1v2 (I/O), io8_166m_ft_fs_pd_1v2 (I/O), io8_166m_ft_ms_1v2 (I/O), io8_166m_ft_ms_pu_1v2 (I/O)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
